| IBIS model for DLPC6401 Controller
[IBIS Ver]   4.0
| Models included herein:
|  DDR2 IO models   DESCRIPTION
|   ZSDDR2DQR   bi-dir IO non-inv., no ODT, no RX power
|  CMOS IO models		DESCRIPTION
| 	bd4stdif		bi-dir IO non-inv.
| 	bd4thdif		bi-dir IO non-inv.
| 	bd8thdif		bi-dir IO non-inv.
| 	bd8thif			bi-dir IO non-inv.
| 	smttdif			input non-inv.
| 	smttif			input non-inv.
| 	smttif_ppd_normal	input non-inv., PCTR=L
| 	smttif_ppd_down		input non-inv., PCTR=H
| 	smttuif			input non-inv.
| 	tlchthdif		input non-inv.
| 	tlchthif_ppd_normal	input non-inv., PCTR=L
| 	tlchthif_ppd_down	input non-inv., PCTR=H
| 	tlchthuif		input non-inv.
| PACKAGE pin models		DESCRIPTION
| 	pbga_package 		DLPC6401
[File name]   dlpc6401control_ibis.ibs
[File Rev]   1.0	| Hideo Oie, first release
[Date]   Nov. 11, 2010
[Source]   DDR2
   HSPICE models used:
   ZSDDR2DQR_rev8.spc Date: 3/10/2010
   CMOS IO Developed by TOSHIBA Corp.
   Package model Developed by Toshiba America Electronic Components
[Notes]   All simulations generated and correlated using HSPICE v2010.03
   C-comp used in all IBIS models is a compromise between on
   (driving) and off (receiving) values. The on (C_comp_on)
   and off (C_comp_off) values have been supplied in the
   model so that they can be used if needed for enhanced
   accuracy.
   Passes ibischk4.2.2 with 0 errors and 27 warnings:
[Disclaimer]	 This information is for modeling purposes only and is not
   guaranteed.
   DDR2 IBIS MODEL HAS BEEN CREATED BY
   s2ibis3 PROCESS. THESE IBIS MODELS ARE PROVIDED "AS IS"
   WITH NO WARRANTY WHATSOEVER AND TOSHIBA SPECIFICALLY
   DISCLAIMS ANY IMPLIED WARRANTIES OF MERCHANTABILITY,
   FITNESS FOR A PARTICULAR PURPOSE, OR AGAINST INFRINGEMENT.
[Copyright]	Copyright(C) Toshiba America Electronics Corporation 2008
 		All rights reserved.
		Copyright(C) TOSHIBA Corp. 1996-2008. All Rights Reserved
[Component] DLPC6401
[Manufacturer]  Toshiba
[Package]
|variable   typ   min   max
R_pkg   734m   NA   NA
L_pkg   6.88nH   NA   NA
C_pkg   1.66pF   NA   NA
[Pin]	signal_name	model_name		R_pin		L_pin		C_pin
M20   AFE_ARSTZ   BT4IF   8.07954e-01   4.14610e-09   1.29491e-12
M21   AFE_CLK   BT8IF   8.55482e-01   4.61930e-09   1.32354e-12
M22   AFE_IRQ   SMTTDIF   9.01286e-01   5.03420e-09   1.26444e-12
N22   ALF_CSYNC   SMTTDIF   9.12752e-01   5.22800e-09   1.29342e-12
P20   ALF_HSYNC   SMTTDIF   8.42291e-01   4.28930e-09   1.30719e-12
P19   ALF_VSYNC   SMTTDIF   7.84877e-01   3.71350e-09   1.29982e-12
J2   CMP_OUT   SMTTIF_PPD_NORMAL   8.73731e-01   4.69920e-09   1.29931e-12
J1   CMP_PWM   BD8THIF   9.04436e-01   4.96420e-09   1.27312e-12
A8   DMD_D0   ZSDDR2DQR   1.00873e+00   5.46140e-09   1.17166e-12
B8   DMD_D1   ZSDDR2DQR   9.65432e-01   5.02080e-09   1.19604e-12
E7   DMD_D10   ZSDDR2DQR   8.81235e-01   3.92900e-09   1.28257e-12
D10   DMD_D11   ZSDDR2DQR   8.72488e-01   3.90170e-09   1.09270e-12
A6   DMD_D12   ZSDDR2DQR   1.04217e+00   5.77030e-09   1.21049e-12
A12   DMD_D13   ZSDDR2DQR   9.97713e-01   5.31100e-09   1.07379e-12
B12   DMD_D14   ZSDDR2DQR   9.53430e-01   4.79680e-09   1.14749e-12
C12   DMD_D15   ZSDDR2DQR   9.10216e-01   4.33350e-09   1.15589e-12
D12   DMD_D16   ZSDDR2DQR   8.69959e-01   3.91470e-09   1.16276e-12
B7   DMD_D17   ZSDDR2DQR   9.85378e-01   5.10680e-09   1.21602e-12
A10   DMD_D18   ZSDDR2DQR   9.93914e-01   5.33470e-09   1.11275e-12
D7   DMD_D19   ZSDDR2DQR   9.02335e-01   4.23820e-09   1.23748e-12
C8   DMD_D2   ZSDDR2DQR   9.37390e-01   4.53740e-09   1.19455e-12
B6   DMD_D20   ZSDDR2DQR   1.00168e+00   5.35160e-09   1.29126e-12
E9   DMD_D21   ZSDDR2DQR   8.54822e-01   3.60610e-09   1.20364e-12
C10   DMD_D22   ZSDDR2DQR   9.14225e-01   4.31530e-09   1.15985e-12
C6   DMD_D23   ZSDDR2DQR   9.55942e-01   4.78070e-09   1.26558e-12
D8   DMD_D3   ZSDDR2DQR   8.99278e-01   4.07110e-09   1.19682e-12
B11   DMD_D4   ZSDDR2DQR   9.52275e-01   4.72750e-09   1.17068e-12
C11   DMD_D5   ZSDDR2DQR   9.11779e-01   4.40350e-09   1.17417e-12
D11   DMD_D6   ZSDDR2DQR   8.71755e-01   3.91570e-09   1.18534e-12
E11   DMD_D7   ZSDDR2DQR   8.32540e-01   3.52120e-09   1.04750e-12
C7   DMD_D8   ZSDDR2DQR   9.47151e-01   4.64830e-09   1.22013e-12
B10   DMD_D9   ZSDDR2DQR   9.55599e-01   4.78170e-09   1.16020e-12
D5   DMD_DAD_BUS   ZSDDR2DQR   8.46083e-01   4.00720e-09   1.29789e-12
B5   DMD_DAD_OEZ   ZSDDR2DQR   9.67753e-01   4.98170e-09   1.28801e-12
C5   DMD_DAD_STRB   ZSDDR2DQR   9.00472e-01   4.46150e-09   1.29938e-12
A9   DMD_DCLK   ZSDDR2DQR   9.98009e-01   5.23180e-09   1.16442e-12
B9   DMD_LOADB   ZSDDR2DQR   9.59740e-01   4.89320e-09   1.17323e-12
G20   DMD_PWR_EN   BD8THIF   8.90199e-01   4.52730e-09   1.33081e-12
D6   DMD_SAC_BUS   ZSDDR2DQR   9.24534e-01   4.40920e-09   1.26132e-12
A5   DMD_SAC_CLK   ZSDDR2DQR   1.02057e+00   5.55180e-09   1.41527e-12
C9   DMD_SCTRL   ZSDDR2DQR   9.19486e-01   4.39700e-09   1.17348e-12
D9   DMD_TRC   ZSDDR2DQR   8.77224e-01   3.93260e-09   1.18082e-12
G3   ETM_PIPESTAT_0  BD8THDIF   8.39283e-01   4.22190e-09   1.34746e-12
G4   ETM_PIPESTAT_1  BD8THDIF   8.27457e-01   4.03920e-09   1.36517e-12
F1   ETM_PIPESTAT_2  BD8THDIF   9.63289e-01   5.50080e-09   1.33587e-12
G2   ETM_TRACECLK   BD8THDIF   8.83028e-01   4.83470e-09   1.35661e-12
F2   ETM_TRACESYNC   BD8THDIF   8.89460e-01   4.80210e-09   1.35839e-12
A3   EXRES   NC | ZSDDR2CALR   8.64776e-01   5.32380e-09   1.77803e-12
H20   EXT_ARSTZ   BT4IF   8.57595e-01   4.48020e-09   1.28194e-12
C15   GPIO_00   BD8THIF   9.26222e-01   4.56720e-09   1.44837e-12
D15   GPIO_01   BD8THIF   8.85806e-01   4.01000e-09   1.33843e-12
A17   GPIO_02   BD8THIF   1.02863e+00   5.72520e-09   1.37065e-12
B16   GPIO_03   BD8THIF   9.86134e-01   5.24710e-09   1.39682e-12
C16   GPIO_04   BD8THIF   9.31786e-01   4.65370e-09   1.36451e-12
D16   GPIO_05   BD8THIF   8.96744e-01   4.19930e-09   1.37755e-12
A18   GPIO_06   BD8THIF   1.00336e+00   5.49550e-09   1.43164e-12
B17   GPIO_07   BD8THIF   9.57989e-01   4.93930e-09   1.40243e-12
J3   GPIO_08   BD8THIF   8.32324e-01   4.18310e-09   1.28634e-12
J4   GPIO_09   BD8THIF   7.92283e-01   3.67520e-09   1.25672e-12
C17   GPIO_10   BD8THIF   9.42340e-01   4.82160e-09   1.34575e-12
A19   GPIO_11   BD8THIF   1.00073e+00   5.45870e-09   1.44411e-12
M4   GPIO_12   BD8THIF   7.69578e-01   3.29580e-09   1.31771e-12
L2   GPIO_13   BD8THIF   9.01499e-01   4.68270e-09   1.24278e-12
B18   GPIO_14   BD8THIF   9.36857e-01   4.94530e-09   1.37659e-12
B19   GPIO_15   BD8THIF   9.44498e-01   5.03630e-09   1.36768e-12
W1   GPIO_16   BD8THIF   8.81846e-01   5.27380e-09   1.33913e-12
V3   GPIO_17   BD8THIF   8.23982e-01   4.21540e-09   1.41644e-12
C18   GPIO_18   BD8THIF   8.98733e-01   4.46560e-09   1.36544e-12
D18   GPIO_19   BD8THIF   8.41460e-01   3.87840e-09   1.32398e-12
N19   GPIO_20   BD8THIF   7.73105e-01   3.67170e-09   1.33610e-12
N20   GPIO_21   BD8THIF   8.20205e-01   4.30190e-09   1.35704e-12
N21   GPIO_22   BD8THIF   8.66684e-01   4.68560e-09   1.37557e-12
D21   GPIO_23   BD8THIF   8.98972e-01   4.82150e-09   1.45690e-12
E20   GPIO_24   BD8THIF   8.74276e-01   4.76150e-09   1.42317e-12
D22   GPIO_25   BD8THIF   9.07763e-01   5.34620e-09   1.47381e-12
F19   GPIO_26   BD8THIF   8.27335e-01   4.27910e-09   1.37653e-12
E21   GPIO_27   BD8THIF   8.86885e-01   4.95580e-09   1.41069e-12
E22   GPIO_28   BD8THIF   8.94467e-01   5.08540e-09   1.44156e-12
F20   GPIO_29   BD8THIF   8.98060e-01   4.66830e-09   1.40455e-12
F21   GPIO_30   BD8THIF   9.46227e-01   5.15500e-09   1.41460e-12
G19   GPIO_31   BD8THIF   8.44715e-01   4.01350e-09   1.39480e-12
F22   GPIO_32   BD8THIF   9.86501e-01   5.65510e-09   1.31127e-12
H2   GPIO_33   BD8THIF   8.87352e-01   4.71450e-09   1.28973e-12
H3   GPIO_34   BD8THIF   8.37248e-01   4.19690e-09   1.32689e-12
H4   GPIO_35   BD8THIF   7.96646e-01   3.82570e-09   1.30908e-12
G1   GPIO_36   BD8THIF   9.26232e-01   5.21610e-09   1.31516e-12
K21   GPIO_37   BD8THIF   8.69314e-01   4.67150e-09   1.23676e-12
V7   HW_TEST_EN   SMTTDIF   8.51026e-01   3.71700e-09   1.24829e-12
V6   ICTSEN   SMTTDIF   8.63167e-01   3.87930e-09   1.23830e-12
M2   IIC0_SCL0   NC | ZSI2CC5L   8.95022e-01   4.40700e-09   1.15987e-12
M3   IIC0_SDA0   NC | ZSI2CC5L   8.96333e-01   4.36760e-09   1.14573e-12
K1   LEDB_EN   BD8THIF   9.26555e-01   4.98450e-09   1.22376e-12
K4   LEDB_PWM   BD8THIF   7.82583e-01   3.62170e-09   1.25673e-12
L4   LEDG_EN   BD8THIF   8.07384e-01   3.77270e-09   1.26227e-12
K3   LEDG_PWM   BD8THIF   8.25593e-01   4.14890e-09   1.22394e-12
L3   LEDR_EN   BD8THIF   8.55421e-01   4.13450e-09   1.27360e-12
K2   LEDR_PWM   BD8THIF   8.71718e-01   4.57700e-09   1.24341e-12
A14   MOSC   NC | OSCIFI   1.07976e+00   5.77890e-09   1.17232e-12
A15   MOSCN   NC | OSCL20IFC1O   1.08111e+00   5.80760e-09   1.25108e-12
AA17   P1_A_0   TLCHTHDIF   9.92652e-01   5.41590e-09   1.38269e-12
W16   P1_A_1   TLCHTHDIF   9.02343e-01   4.25710e-09   1.42080e-12
AB18   P1_A_2   TLCHTHDIF   1.01157e+00   5.71520e-09   1.43592e-12
Y17   P1_A_3   TLCHTHDIF   9.46887e-01   4.94000e-09   1.36731e-12
AA18   P1_A_4   TLCHTHDIF   9.74621e-01   5.24930e-09   1.45887e-12
AB19   P1_A_5   TLCHTHDIF   9.84595e-01   5.54790e-09   1.66377e-12
W17   P1_A_6   TLCHTHDIF   8.94120e-01   4.33450e-09   1.47509e-12
Y18   P1_A_7   TLCHTHDIF   9.07907e-01   4.67210e-09   1.37447e-12
AA19   P1_A_8   TLCHTHDIF   9.52112e-01   5.27560e-09   1.48397e-12
AB20   P1_A_9   TLCHTHDIF   9.70798e-01   5.75090e-09   1.77457e-12
W18   P1_B_0   TLCHTHDIF   7.89869e-01   3.76450e-09   1.39067e-12
Y19   P1_B_1   TLCHTHDIF   8.42812e-01   4.49200e-09   1.46088e-12
AA20   P1_B_2   TLCHTHDIF   8.73819e-01   4.94660e-09   1.63951e-12
W21   P1_B_3   TLCHTHDIF   9.17206e-01   4.98260e-09   1.32707e-12
W22   P1_B_4   TLCHTHDIF   9.25681e-01   5.21260e-09   1.45852e-12
V21   P1_B_5   TLCHTHDIF   9.14758e-01   4.82460e-09   1.25065e-12
U19   P1_B_6   TLCHTHDIF   8.63957e-01   4.18160e-09   1.33835e-12
V22   P1_B_7   TLCHTHDIF   9.17072e-01   5.00740e-09   1.61320e-12
U20   P1_B_8   TLCHTHDIF   8.80951e-01   4.46250e-09   1.35318e-12
U21   P1_B_9   TLCHTHDIF   9.36798e-01   5.06510e-09   1.36980e-12
U22   P1_C_0   TLCHTHDIF   9.48174e-01   5.23980e-09   1.27272e-12
T19   P1_C_1   TLCHTHDIF   8.43580e-01   3.95220e-09   1.25345e-12
T20   P1_C_2   TLCHTHDIF   8.80183e-01   4.44640e-09   1.28649e-12
T21   P1_C_3   TLCHTHDIF   9.24713e-01   4.91180e-09   1.29547e-12
R22   P1_C_4   TLCHTHDIF   9.60692e-01   5.27580e-09   1.28910e-12
R21   P1_C_5   TLCHTHDIF   9.16424e-01   4.89350e-09   1.33117e-12
R20   P1_C_6   TLCHTHDIF   8.77324e-01   4.41810e-09   1.27723e-12
R19   P1_C_7   TLCHTHDIF   8.28149e-01   3.81180e-09   1.26699e-12
P22   P1_C_8   TLCHTHDIF   9.13476e-01   5.28510e-09   1.28922e-12
P21   P1_C_9   TLCHTHDIF   8.85451e-01   4.74100e-09   1.34492e-12
AA16   P1_DATEN   TLCHTHDIF   1.00033e+00   5.28570e-09   1.40104e-12
W14   P1_FIELD   TLCHTHDIF   8.88291e-01   3.87980e-09   1.37421e-12
AB16   P1_HSYNC   BD4THDIF   1.03775e+00   5.65570e-09   1.30817e-12
Y15   P1_VSYNC   BD4STDIF   9.45882e-01   4.59550e-09   1.31167e-12
W15   P1A_CLK   TLCHTHDIF   9.00073e-01   4.26010e-09   1.42529e-12
AB17   P1B_CLK   TLCHTHDIF   1.04769e+00   5.91140e-09   1.39382e-12
Y16   P1C_CLK   TLCHTHDIF   9.47628e-01   4.72320e-09   1.35816e-12
D13   PLLD_VAD   NC | ZSAPLVDAC5L   8.41797e-01   3.82040e-09   1.22002e-12
C13   PLLD_VAS   NC | ZSAPLVSAC5L   8.48949e-01   4.01310e-09   1.15124e-12
E13   PLLD_VDD   NC | ZSAPLVDDC5L   6.49781e-01   2.68610e-09   1.34973e-12
B14   PLLD_VSS   NC | ZSAPLVSDC5L   9.02685e-01   4.89560e-09   1.44556e-12
D14   PLLM_VAD   NC | ZSAPLVDAC5L   8.51564e-01   3.94730e-09   3.82711e-12
C14   PLLM_VAS   NC | ZSAPLVSAC5L   8.78515e-01   4.33480e-09   1.39565e-12
E14   PLLM_VDD   NC | ZSAPLVDDC5L   8.29996e-01   3.56460e-09   1.21975e-12
B15   PLLM_VSS   NC | ZSAPLVSDC5L   9.24921e-01   4.90080e-09   1.45306e-12
AB7   PM_ADDR_00   BT8IF   1.02438e+00   5.81800e-09   1.34538e-12
AA7   PM_ADDR_01   BT8IF   9.79168e-01   5.20980e-09   1.36026e-12
W8   PM_ADDR_02   BT8IF   8.81413e-01   4.09600e-09   1.36950e-12
AB6   PM_ADDR_03   BT8IF   1.03327e+00   5.93930e-09   1.32781e-12
Y7   PM_ADDR_04   BT8IF   9.35480e-01   4.69310e-09   1.38190e-12
AA6   PM_ADDR_05   BT8IF   9.59757e-01   4.97880e-09   1.41213e-12
AB5   PM_ADDR_06   BT8IF   1.00505e+00   5.53160e-09   1.57933e-12
W7   PM_ADDR_07   BT8IF   8.98241e-01   4.24300e-09   1.34658e-12
Y6   PM_ADDR_08   BT8IF   9.15788e-01   4.56920e-09   1.39972e-12
AA5   PM_ADDR_09   BT8IF   9.89108e-01   5.39020e-09   1.45766e-12
AB4   PM_ADDR_10   BT8IF   1.01300e+00   5.85560e-09   1.46435e-12
W6   PM_ADDR_11   BT8IF   9.28171e-01   4.48060e-09   1.48290e-12
Y5   PM_ADDR_12   BT8IF   9.43399e-01   4.79100e-09   1.50231e-12
AA4   PM_ADDR_13   BT8IF   9.92652e-01   5.40050e-09   1.68348e-12
AB3   PM_ADDR_14   BT8IF   1.03690e+00   6.18410e-09   1.56178e-12
W5   PM_ADDR_15   BT8IF   8.97752e-01   4.15450e-09   1.46612e-12
Y4   PM_ADDR_16   BT8IF   9.29585e-01   4.72250e-09   1.57453e-12
AA3   PM_ADDR_17   BT8IF   9.94863e-01   5.59320e-09   1.40757e-12
AB2   PM_ADDR_18   BT8IF   1.00373e+00   5.69490e-09   1.80759e-12
Y1   PM_ADDR_19   BT8IF   8.95475e-01   5.04070e-09   1.56249e-12
W2   PM_ADDR_20   BT8IF   8.71686e-01   4.86130e-09   1.36991e-12
AB8   PM_BLSZ_0   BT8IF   9.70385e-01   4.92060e-09   1.34491e-12
AA8   PM_BLSZ_1   BT8IF   9.31170e-01   4.63110e-09   1.36414e-12
U3   PM_CSZ_0   BT8IF   8.84811e-01   4.74780e-09   1.37040e-12
U2   PM_CSZ_1   BT8IF   9.23568e-01   5.15160e-09   1.45081e-12
U1   PM_CSZ_2   BT8IF   9.64906e-01   5.60130e-09   1.36416e-12
T4   PM_DATA_00   BD8THIF   8.20528e-01   4.06540e-09   1.35226e-12
T3   PM_DATA_01   BD8THIF   8.68318e-01   4.58780e-09   1.37082e-12
T2   PM_DATA_02   BD8THIF   9.11001e-01   4.99600e-09   1.42562e-12
T1   PM_DATA_03   BD8THIF   9.56027e-01   5.59720e-09   1.32654e-12
R4   PM_DATA_04   BD8THIF   8.19550e-01   4.01020e-09   1.40400e-12
R3   PM_DATA_05   BD8THIF   8.69795e-01   4.62620e-09   1.37352e-12
R2   PM_DATA_06   BD8THIF   9.09879e-01   4.99840e-09   1.28176e-12
P4   PM_DATA_07   BD8THIF   8.11209e-01   3.79770e-09   1.27544e-12
P3   PM_DATA_08   BD8THIF   8.65388e-01   4.38040e-09   1.29546e-12
P2   PM_DATA_09   BD8THIF   9.06151e-01   4.86000e-09   1.31845e-12
P1   PM_DATA_10   BD8THIF   9.56301e-01   5.35330e-09   1.28033e-12
N4   PM_DATA_11   BD8THIF   8.10852e-01   3.75880e-09   1.31589e-12
N3   PM_DATA_12   BD8THIF   8.58045e-01   4.30580e-09   1.30065e-12
N2   PM_DATA_13   BD8THIF   9.02433e-01   4.84640e-09   1.33875e-12
N1   PM_DATA_14   BD8THIF   9.39943e-01   5.20810e-09   1.26949e-12
M1   PM_DATA_15   BD8THIF   9.09485e-01   4.97960e-09   1.25476e-12
U4   PM_OEZ   BT8IF   8.40007e-01   4.17660e-09   1.32304e-12
V2   PM_WEZ   BT8IF   8.69487e-01   4.76480e-09   1.27612e-12
G21   POSENSE   SMTTIF   9.41247e-01   4.99470e-09   1.31840e-12
H19   PWRGOOD   SMTTIF_PPD_NORMAL   8.43319e-01   3.95090e-09   1.25086e-12
AA10   RA_IN_N   ZEFPDL_N_V33   9.98970e-01   4.88360e-09   1.26394e-12
AB10   RA_IN_P   ZEFPDL_P_V33   9.98481e-01   4.95230e-09   1.24464e-12
W11   RB_IN_N   ZEFPDL_N_V33   8.87198e-01   3.96060e-09   1.25427e-12
Y11   RB_IN_P   ZEFPDL_P_V33   8.85266e-01   3.81520e-09   1.23058e-12
AA12   RC_IN_N   ZEFPDL_N_V33   9.80596e-01   4.75100e-09   1.23859e-12
AB12   RC_IN_P   ZEFPDL_P_V33   9.84972e-01   4.75820e-09   1.19848e-12
W9   RCK_IN_N   ZEFPDL_N_V33   9.13662e-01   4.08620e-09   1.34463e-12
Y9   RCK_IN_P   ZEFPDL_P_V33   9.15145e-01   4.17470e-09   1.30690e-12
W13   RD_IN_N   ZEFPDL_N_V33   8.89470e-01   3.93810e-09   1.23364e-12
Y13   RD_IN_P   ZEFPDL_P_V33   8.92889e-01   3.87020e-09   1.23888e-12
AA14   RE_IN_N   ZEFPDL_N_V33   9.99469e-01   4.85940e-09   1.25980e-12
AB14   RE_IN_P   ZEFPDL_P_V33   1.00448e+00   4.95400e-09   1.23269e-12
G18   RTCK   BT8IF   8.18892e-01   3.85830e-09   1.50638e-12
E16   SPARE_3   BD8THIF   8.53124e-01   3.68740e-09   1.37655e-12
F4   SSP0_CLK   BD8THIF   8.29766e-01   4.20870e-09   1.45567e-12
D2   SSP0_CSZ_0   BD8THIF   8.48081e-01   4.79560e-09   1.40818e-12
C1   SSP0_CSZ_1   BD8THIF   8.71202e-01   5.23480e-09   1.63427e-12
D1   SSP0_RXD   TLCHTHIF_PPD_NORMAL  9.30363e-01   5.64140e-09   1.54423e-12
F3   SSP0_TXD   BT8IF   8.59525e-01   4.45270e-09   1.35345e-12
R18   TCK   TLCHTHUIF   7.57224e-01   3.53830e-09   1.40358e-12
P18   TDI   TLCHTHUIF   7.44901e-01   3.36920e-09   1.35220e-12
L18   TDO1   BT4IF   7.38478e-01   3.25620e-09   1.37627e-12
M18   TDO2   BT4IF   7.75898e-01   3.95130e-09   1.37712e-12
V15   TMS1   TLCHTHUIF   8.57527e-01   3.75030e-09   1.43530e-12
V16   TMS2   TLCHTHUIF   8.57453e-01   3.83660e-09   1.34509e-12
V17   TRSTZ   SMTTUIF   8.19065e-01   3.70880e-09   1.33217e-12
H21   TSTPT_0   BD8THDIF   9.02414e-01   4.85340e-09   1.29200e-12
H22   TSTPT_1   BD8THDIF   9.36795e-01   5.37530e-09   1.27649e-12
J19   TSTPT_2   BD8THDIF   7.94154e-01   3.71050e-09   1.32727e-12
J20   TSTPT_3   BD8THDIF   8.37688e-01   4.27830e-09   1.30602e-12
J21   TSTPT_4   BD8THDIF   8.80095e-01   4.80930e-09   1.32968e-12
J22   TSTPT_5   BD8THDIF   9.25963e-01   5.29630e-09   1.28487e-12
K19   TSTPT_6   BD8THDIF   7.82631e-01   3.63900e-09   1.27063e-12
K20   TSTPT_7   BD8THDIF   8.27665e-01   4.15010e-09   1.26995e-12
L20   UART0_CTSZ   TLCHTHIF_PPD_NORMAL  8.20252e-01   4.09100e-09   1.26162e-12
M19   UART0_RTSZ   BT8IF   7.78295e-01   3.64320e-09   1.26933e-12
L21   UART0_RXD   TLCHTHIF_PPD_NORMAL  8.63187e-01   4.60420e-09   1.29825e-12
L19   UART0_TXD   BT8IF   7.82345e-01   3.65830e-09   1.25517e-12
E3   USB_DAT_N   NC | ZSUSBDDRV33C5L   9.10488e-01   4.77270e-09   1.31033e-12
E2   USB_DAT_P   NC | ZSUSBDDRV33C5L   9.14545e-01   4.88180e-09   1.33738e-12
D17   VPGM   NC | DIPLSHVR33_VPGM   8.62424e-01   4.19740e-09   1.35531e-12
F13 	 PG9   NC | NA   NA   NA   NA
[Package Model] pbga_package
|   Model SMTTIF_PPD
[Model Selector] SMTTIF_PPD
SMTTIF_PPD_NORMAL   PCTR=L
SMTTIF_PPD_DOWN   PCTR=H
|   Model TLCHTHIF_PPD
[Model Selector] tlchthif_ppd
TLCHTHIF_PPD_NORMAL   PCTR=L
TLCHTHIF_PPD_DOWN   PCTR=H
[Define Package Model]  pbga_package
[Manufacturer]   Toshiba
[OEM]   unknown
[Description]   DPP6401
[Number Of Pins]   232
[Pin Numbers]
M20 | 1 BGA-M20 AFE_ARSTZ
M21 | 2 BGA-M21 AFE_CLK
M22 | 3 BGA-M22 AFE_IRQ
N19 | 4 BGA-N19 GPIO_20
N20 | 5 BGA-N20 GPIO_21
N21 | 6 BGA-N21 GPIO_22
L18 | 7 BGA-L18 TDO1
M18 | 8 BGA-M18 TDO2
L20 | 9 BGA-L20 UART0_CTSZ
M19 | 10 BGA-M19 UART0_RTSZ
L21 | 11 BGA-L21 UART0_RXD
L19 | 12 BGA-L19 UART0_TXD
N22 | 13 BGA-N22 ALF_CSYNC
P18 | 14 BGA-P18 TDI
P20 | 15 BGA-P20 ALF_HSYNC
P19 | 16 BGA-P19 ALF_VSYNC
P22 | 17 BGA-P22 P1_C_8
P21 | 18 BGA-P21 P1_C_9
R21 | 19 BGA-R21 P1_C_5
R20 | 20 BGA-R20 P1_C_6
R19 | 21 BGA-R19 P1_C_7
R18 | 22 BGA-R18 TCK
J2 | 23 BGA-J2 CMP_OUT
J1 | 24 BGA-J1 CMP_PWM
J3 | 25 BGA-J3 GPIO_08
J4 | 26 BGA-J4 GPIO_09
H2 | 27 BGA-H2 GPIO_33
H3 | 28 BGA-H3 GPIO_34
H4 | 29 BGA-H4 GPIO_35
G1 | 30 BGA-G1 GPIO_36
K1 | 31 BGA-K1 LEDB_EN
K4 | 32 BGA-K4 LEDB_PWM
L4 | 33 BGA-L4 LEDG_EN
K3 | 34 BGA-K3 LEDG_PWM
K2 | 35 BGA-K2 LEDR_PWM
A8 | 36 BGA-A8 DMD_D0
B8 | 37 BGA-B8 DMD_D1
D10 | 38 BGA-D10 DMD_D11
B7 | 39 BGA-B7 DMD_D17
C8 | 40 BGA-C8 DMD_D2
E9 | 41 BGA-E9 DMD_D21
D8 | 42 BGA-D8 DMD_D3
C7 | 43 BGA-C7 DMD_D8
A9 | 44 BGA-A9 DMD_DCLK
B9 | 45 BGA-B9 DMD_LOADB
C9 | 46 BGA-C9 DMD_SCTRL
D9 | 47 BGA-D9 DMD_TRC
E7 | 48 BGA-E7 DMD_D10
A6 | 49 BGA-A6 DMD_D12
D7 | 50 BGA-D7 DMD_D19
B6 | 51 BGA-B6 DMD_D20
C6 | 52 BGA-C6 DMD_D23
D5 | 53 BGA-D5 DMD_DAD_BUS
B5 | 54 BGA-B5 DMD_DAD_OEZ
C5 | 55 BGA-C5 DMD_DAD_STRB
D6 | 56 BGA-D6 DMD_SAC_BUS
A5 | 57 BGA-A5 DMD_SAC_CLK
A10 | 58 BGA-A10 DMD_D18
C10 | 59 BGA-C10 DMD_D22
B11 | 60 BGA-B11 DMD_D4
C11 | 61 BGA-C11 DMD_D5
D11 | 62 BGA-D11 DMD_D6
E11 | 63 BGA-E11 DMD_D7
B10 | 64 BGA-B10 DMD_D9
A12 | 65 BGA-A12 DMD_D13
B12 | 66 BGA-B12 DMD_D14
C12 | 67 BGA-C12 DMD_D15
D12 | 68 BGA-D12 DMD_D16
A14 | 69 BGA-A14 MOSC
A15 | 70 BGA-A15 MOSCN
F13 | 71 BGA-F13 PG9
D13 | 72 BGA-D13 PLLD_VAD
C13 | 73 BGA-C13 PLLD_VAS
E13 | 74 BGA-E13 PLLD_VDD
A3 | 75 BGA-A3 EXRES
G20 | 76 BGA-G20 DMD_PWR_EN
H20 | 77 BGA-H20 EXT_ARSTZ
E21 | 78 BGA-E21 GPIO_27
E22 | 79 BGA-E22 GPIO_28
F20 | 80 BGA-F20 GPIO_29
F21 | 81 BGA-F21 GPIO_30
G19 | 82 BGA-G19 GPIO_31
F22 | 83 BGA-F22 GPIO_32
G21 | 84 BGA-G21 POSENSE
H19 | 85 BGA-H19 PWRGOOD
G18 | 86 BGA-G18 RTCK
H21 | 87 BGA-H21 TSTPT_0
H22 | 88 BGA-H22 TSTPT_1
J19 | 89 BGA-J19 TSTPT_2
G3 | 90 BGA-G3 ETM_PIPESTAT_0
G4 | 91 BGA-G4 ETM_PIPESTAT_1
F1 | 92 BGA-F1 ETM_PIPESTAT_2
G2 | 93 BGA-G2 ETM_TRACECLK
F2 | 94 BGA-F2 ETM_TRACESYNC
F4 | 95 BGA-F4 SSP0_CLK
D1 | 96 BGA-D1 SSP0_RXD
F3 | 97 BGA-F3 SSP0_TXD
E3 | 98 BGA-E3 USB_DAT_N
E2 | 99 BGA-E2 USB_DAT_P
C1 | 100 BGA-C1 SSP0_CSZ_1
J20 | 101 BGA-J20 TSTPT_3
J21 | 102 BGA-J21 TSTPT_4
C15 | 103 BGA-C15 GPIO_00
D15 | 104 BGA-D15 GPIO_01
A17 | 105 BGA-A17 GPIO_02
B16 | 106 BGA-B16 GPIO_03
C16 | 107 BGA-C16 GPIO_04
D16 | 108 BGA-D16 GPIO_05
B14 | 109 BGA-B14 PLLD_VSS
D14 | 110 BGA-D14 PLLM_VAD
C14 | 111 BGA-C14 PLLM_VAS
E14 | 112 BGA-E14 PLLM_VDD
B15 | 113 BGA-B15 PLLM_VSS
E16 | 114 BGA-E16 SPARE_3
A18 | 115 BGA-A18 GPIO_06
B17 | 116 BGA-B17 GPIO_07
C17 | 117 BGA-C17 GPIO_10
D18 | 118 BGA-D18 GPIO_19
D17 | 119 BGA-D17 VPGM
A19 | 120 BGA-A19 GPIO_11
B18 | 121 BGA-B18 GPIO_14
C18 | 122 BGA-C18 GPIO_18
B19 | 123 BGA-B19 GPIO_15
M4 | 124 BGA-M4 GPIO_12
L2 | 125 BGA-L2 GPIO_13
M2 | 126 BGA-M2 IIC0_SCL0
M3 | 127 BGA-M3 IIC0_SDA0
L3 | 128 BGA-L3 LEDR_EN
P2 | 129 BGA-P2 PM_DATA_09
P1 | 130 BGA-P1 PM_DATA_10
N4 | 131 BGA-N4 PM_DATA_11
N3 | 132 BGA-N3 PM_DATA_12
N2 | 133 BGA-N2 PM_DATA_13
N1 | 134 BGA-N1 PM_DATA_14
M1 | 135 BGA-M1 PM_DATA_15
W1 | 136 BGA-W1 GPIO_16
V3 | 137 BGA-V3 GPIO_17
Y1 | 138 BGA-Y1 PM_ADDR_19
W2 | 139 BGA-W2 PM_ADDR_20
U3 | 140 BGA-U3 PM_CSZ_0
T4 | 141 BGA-T4 PM_DATA_00
U4 | 142 BGA-U4 PM_OEZ
V2 | 143 BGA-V2 PM_WEZ
U2 | 144 BGA-U2 PM_CSZ_1
U1 | 145 BGA-U1 PM_CSZ_2
D21 | 146 BGA-D21 GPIO_23
E20 | 147 BGA-E20 GPIO_24
D22 | 148 BGA-D22 GPIO_25
F19 | 149 BGA-F19 GPIO_26
K21 | 150 BGA-K21 GPIO_37
J22 | 151 BGA-J22 TSTPT_5
K19 | 152 BGA-K19 TSTPT_6
K20 | 153 BGA-K20 TSTPT_7
V7 | 154 BGA-V7 HW_TEST_EN
V6 | 155 BGA-V6 ICTSEN
AB7 | 156 BGA-AB7 PM_ADDR_00
AA7 | 157 BGA-AA7 PM_ADDR_01
W8 | 158 BGA-W8 PM_ADDR_02
AB6 | 159 BGA-AB6 PM_ADDR_03
Y7 | 160 BGA-Y7 PM_ADDR_04
AA6 | 161 BGA-AA6 PM_ADDR_05
AB5 | 162 BGA-AB5 PM_ADDR_06
W7 | 163 BGA-W7 PM_ADDR_07
Y6 | 164 BGA-Y6 PM_ADDR_08
AA5 | 165 BGA-AA5 PM_ADDR_09
AB4 | 166 BGA-AB4 PM_ADDR_10
W6 | 167 BGA-W6 PM_ADDR_11
Y5 | 168 BGA-Y5 PM_ADDR_12
AA4 | 169 BGA-AA4 PM_ADDR_13
AB3 | 170 BGA-AB3 PM_ADDR_14
W5 | 171 BGA-W5 PM_ADDR_15
Y4 | 172 BGA-Y4 PM_ADDR_16
AA3 | 173 BGA-AA3 PM_ADDR_17
AB2 | 174 BGA-AB2 PM_ADDR_18
AB8 | 175 BGA-AB8 PM_BLSZ_0
AA8 | 176 BGA-AA8 PM_BLSZ_1
AA17 | 177 BGA-AA17 P1_A_0
W16 | 178 BGA-W16 P1_A_1
AB18 | 179 BGA-AB18 P1_A_2
Y17 | 180 BGA-Y17 P1_A_3
AA18 | 181 BGA-AA18 P1_A_4
AB19 | 182 BGA-AB19 P1_A_5
W17 | 183 BGA-W17 P1_A_6
Y18 | 184 BGA-Y18 P1_A_7
AA16 | 185 BGA-AA16 P1_DATEN
AB16 | 186 BGA-AB16 P1_HSYNC
Y15 | 187 BGA-Y15 P1_VSYNC
W15 | 188 BGA-W15 P1A_CLK
AB17 | 189 BGA-AB17 P1B_CLK
Y16 | 190 BGA-Y16 P1C_CLK
V15 | 191 BGA-V15 TMS1
V16 | 192 BGA-V16 TMS2
V17 | 193 BGA-V17 TRSTZ
AA19 | 194 BGA-AA19 P1_A_8
W14 | 195 BGA-W14 P1_FIELD
AB20 | 196 BGA-AB20 P1_A_9
W18 | 197 BGA-W18 P1_B_0
Y19 | 198 BGA-Y19 P1_B_1
AA20 | 199 BGA-AA20 P1_B_2
W21 | 200 BGA-W21 P1_B_3
W22 | 201 BGA-W22 P1_B_4
V21 | 202 BGA-V21 P1_B_5
U19 | 203 BGA-U19 P1_B_6
V22 | 204 BGA-V22 P1_B_7
U20 | 205 BGA-U20 P1_B_8
T19 | 206 BGA-T19 P1_C_1
U21 | 207 BGA-U21 P1_B_9
U22 | 208 BGA-U22 P1_C_0
T20 | 209 BGA-T20 P1_C_2
T21 | 210 BGA-T21 P1_C_3
R22 | 211 BGA-R22 P1_C_4
AB14 | 212 BGA-AB14 RE_IN_P
W13 | 213 BGA-W13 RD_IN_N
Y13 | 214 BGA-Y13 RD_IN_P
AA14 | 215 BGA-AA14 RE_IN_N
W9 | 216 BGA-W9 RCK_IN_N
Y9 | 217 BGA-Y9 RCK_IN_P
T3 | 218 BGA-T3 PM_DATA_01
T2 | 219 BGA-T2 PM_DATA_02
R4 | 220 BGA-R4 PM_DATA_04
T1 | 221 BGA-T1 PM_DATA_03
R3 | 222 BGA-R3 PM_DATA_05
P4 | 223 BGA-P4 PM_DATA_07
R2 | 224 BGA-R2 PM_DATA_06
P3 | 225 BGA-P3 PM_DATA_08
AA10 | 226 BGA-AA10 RA_IN_N
AB10 | 227 BGA-AB10 RA_IN_P
W11 | 228 BGA-W11 RB_IN_N
Y11 | 229 BGA-Y11 RB_IN_P
AA12 | 230 BGA-AA12 RC_IN_N
AB12 | 231 BGA-AB12 RC_IN_P
D2 | 232 BGA-D2 SSP0_CSZ_0
[Model Data]
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[End Model Data]
[End Package Model]
| Models and submodels in the file (18): ZEFPDL_P_V33 (Input), ZEFPDL_N_V33 (Input), BD4STDIF (I/O), BD4THDIF (I/O), BD8THDIF (I/O), BD8THIF (I/O), BT4IF (3-state), BT8IF (3-state), SMTTDIF (Input), SMTTIF (Input), SMTTIF_PPD_NORMAL (Input), SMTTIF_PPD_DOWN (Input), SMTTUIF (Input), TLCHTHDIF (Input), TLCHTHIF_PPD_NORMAL (Input), TLCHTHIF_PPD_DOWN (Input), TLCHTHUIF (Input), ZSDDR2DQR (I/O)
